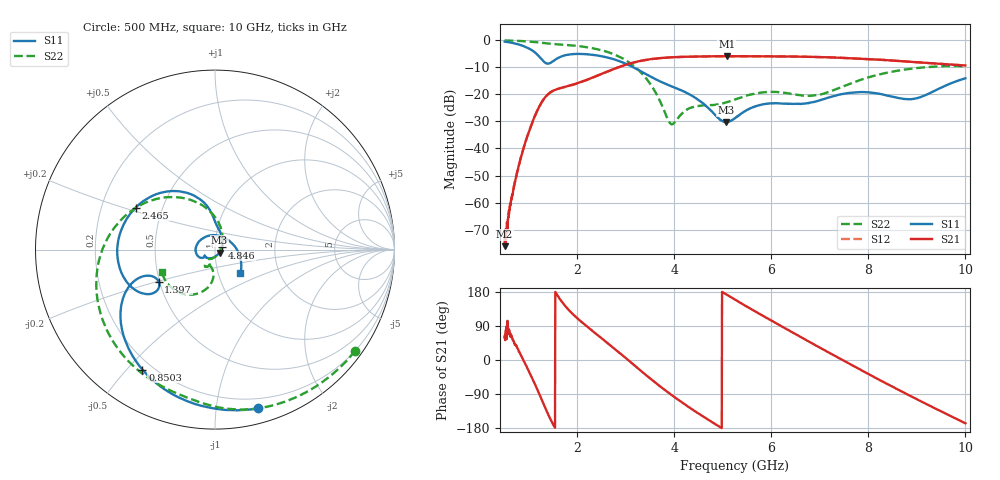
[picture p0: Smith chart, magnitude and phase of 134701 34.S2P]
!  2-Port S-parameters saved by WinCal
! VAR MeasName=S-Parameters (CALIBRATED_DATA) read from VNA (N5242A)
! VAR MeasDate=2013-7-3 16:36:33
! VAR NAME=134701 34
! VAR FILENAME=134701 34.S2P
! VAR DATE=2013-7-3 16:36:33
! VAR PHYS_PORTS=1,2
# Hz S MA R 50
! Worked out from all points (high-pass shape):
!   1601 points, 500 MHz to 10 GHz, reference 50 ohm
!   highest |S21| = -6.12 dB at 5.078 GHz (marker M1); lowest = -76.0 dB at 500 MHz (marker M2)
!   |S21| within 3 dB of the highest: 3.027 GHz to 9.632 GHz (6.605 GHz wide, 104 % of centre)
!   lowest |S11| = -30.5 dB at 5.06 GHz (marker M3), VSWR 1.06, Z = 52.5 - j1.71 ohm
!   |S11| at or under -10 dB: 3.131 GHz to end of sweep
!   |S22| runs from -31.2 to -0.3 dB; largest |S21 - S12| = 0.0021
!   S11 on the Smith chart (normalised r, x): 500 MHz: 0.12, -1.30; 850.3 MHz: 0.16, -0.55; 1.397 GHz: 0.49, -0.20; 2.465 GHz: 0.35, +0.22; 4.846 GHz: 1.08, +0.03; 10 GHz: 1.28, -0.35
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5e8  0.917 -74.8  0.0001588 59.6  0.000249 86.9  0.963 -35.9
6.603125e8  0.8688 -96.7  0.001414 56.5  0.001372 58.8  0.9533 -47.2
8.503125e8  0.7815 -121.1  0.007528 9.6  0.007574 8.7  0.9387 -60.7
1.194688e9  0.5078 -157.6  0.05403 -83.8  0.05401 -84.1  0.89 -85.3
1.396562e9  0.361 -150.4  0.09891 -143.2  0.0988 -143.5  0.845 -98.5
1.657812e9  0.4843 -150.6  0.1286 157.4  0.1281 157.2  0.8103 -114.9
2.085312e9  0.544 178.4  0.1675 100.2  0.1667 100.1  0.7471 -144.8
2.465312e9  0.5001 152.0  0.2274 60.9  0.2261 60.9  0.6486 -174.8
3.0175e9  0.3531 116.4  0.3484 3.0  0.3475 3.2  0.4067 134.5
3.670625e9  0.1763 92.4  0.4539 -66.2  0.4529 -66.1  0.08517 60.2
3.949688e9  0.137 86.5  0.4721 -93.1  0.4718 -93.1  0.02753 -30.9
4.311875e9  0.09814 71.7  0.4849 -125.4  0.4849 -125.4  0.05481 -110.2
4.84625e9  0.04055 17.7  0.4935 -169.5  0.4934 -169.4  0.06324 -118.2
5.06e9  0.02992 -32.9  0.4939 173.8  0.4945 173.8  0.06976 -112.8
5.077812e9  0.03026 -37.9  0.4945 172.4  0.4944 172.4  0.07034 -112.2
5.25e9  0.03594 -77.8  0.4942 159.2  0.4945 159.2  0.07938 -109.7
6.063438e9  0.06746 -144.4  0.4905 99.4  0.4906 99.5  0.109 -120.2
6.835312e9  0.06998 -146.4  0.481 44.2  0.4813 44.2  0.09306 -110.9
7.55375e9  0.1027 -160.3  0.4574 -6.3  0.4575 -6.4  0.1457 -93.4
8.420625e9  0.09231 136.4  0.4162 -65.6  0.4147 -65.6  0.2491 -108.1
8.984688e9  0.08271 56.4  0.3843 -102.5  0.383 -102.6  0.2984 -123.7
1e10  0.1942 -43.1  0.3343 -167.0  0.3339 -166.8  0.321 -156.7
